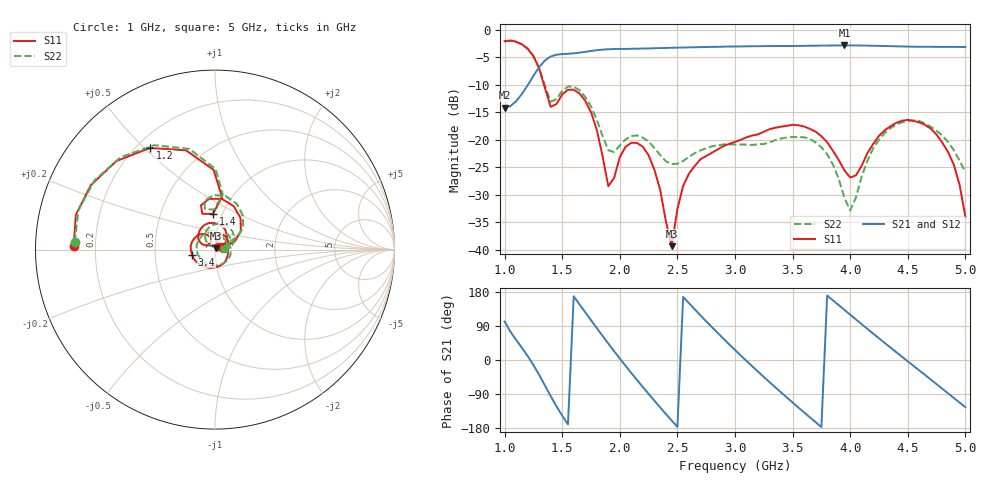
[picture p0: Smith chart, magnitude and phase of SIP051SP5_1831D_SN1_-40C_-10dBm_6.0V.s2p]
# GHz  S  dB  R  50
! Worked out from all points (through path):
!   81 points, 1 GHz to 5 GHz, reference 50 ohm
!   highest |S21| = -2.84 dB at 3.95 GHz (marker M1); lowest = -14.1 dB at 1 GHz (marker M2)
!   lowest |S11| = -39.3 dB at 2.45 GHz (marker M3), VSWR 1.02, Z = 50.7 + j0.828 ohm
!   |S11| at or under -10 dB: 1.342 GHz to end of sweep
!   |S22| runs from -32.8 to -2.0 dB; largest |S21 - S12| = 0.0022
!   S11 on the Smith chart (normalised r, x): 1 GHz: 0.12, +0.01; 1.2 GHz: 0.25, +0.52; 1.4 GHz: 0.90, +0.38; 3.4 GHz: 0.77, -0.04; 5 GHz: 1.03, +0.03
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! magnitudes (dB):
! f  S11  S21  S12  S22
! 1 GHz  -2.1  -14.1  -14.2  -2.1
! 1.2 GHz  -3.4  -10.1  -10.1  -3.4
! 1.4 GHz  -14.0  -4.9  -4.9  -13.1
! 1.55 GHz  -10.9  -4.4  -4.4  -10.3
! 1.7 GHz  -12.9  -4.0  -4.0  -12.2
! 1.8 GHz  -18.2  -3.7  -3.7  -16.3
! 1.9 GHz  -28.4  -3.5  -3.5  -21.9
! 2.05 GHz  -21.3  -3.5  -3.5  -19.9
! 2.15 GHz  -20.6  -3.4  -3.4  -19.2
! 2.35 GHz  -29.0  -3.3  -3.3  -22.8
! 2.45 GHz  -39.3  -3.3  -3.3  -24.4
! 2.6 GHz  -26.2  -3.2  -3.2  -23.1
! 3 GHz  -20.4  -3.0  -3.0  -20.8
! 3.4 GHz  -17.6  -3.0  -2.9  -19.8
! 3.7 GHz  -18.5  -2.9  -2.9  -20.5
! 3.95 GHz  -25.5  -2.8  -2.8  -30.5
! 4 GHz  -26.8  -2.9  -2.9  -32.8
! 4.2 GHz  -20.7  -2.9  -2.9  -21.5
! 4.35 GHz  -17.5  -3.0  -3.0  -17.9
! 4.75 GHz  -19.1  -3.1  -3.1  -18.4
! 4.9 GHz  -24.6  -3.1  -3.1  -21.9
! 5 GHz  -34.0  -3.1  -3.2  -25.8
